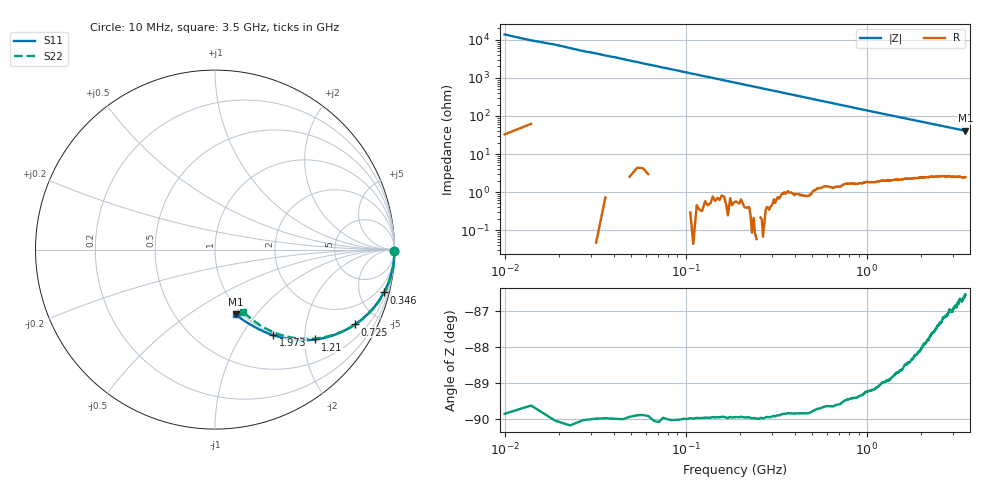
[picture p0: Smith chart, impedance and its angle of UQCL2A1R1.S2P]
! AVX Corporation
! Date:  10/27/06
! Part No:  UQCL2A1R1
! Description:  Ultra Low ESR Microwave capacitors
! Mounting Orientation:  Horizontal
# GHZ S DB R 50
! Freq  |S11|  S11 Ph  |S21|  S21 Ph  |S12|  S12 Ph  |S22|  S22 Ph
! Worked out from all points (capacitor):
!   801 points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, 10 MHz to 3.5 GHz, reference 50 ohm
!   read as one part in series: C = 1.13 pF near 27 MHz
!   lowest |Z| = 40.9 ohm at 3.5 GHz (marker M1)
!   S11 on the Smith chart (normalised r, x): 10 MHz: open; 346 MHz: 0.96, -7.89; 725 MHz: 0.98, -3.76; 1.21 GHz: 0.98, -2.25; 1.973 GHz: 0.98, -1.39; 3.5 GHz: 0.94, -0.79
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0.01  -0.01 -0.3  -42.87 89.5  -42.77 89.8  -0.01 -0.5
0.019  -0.01 -0.8  -37.53 89.3  -37.50 89.0  -0.01 -0.8
0.036  -0.01 -1.6  -31.81 88.4  -31.79 88.5  -0.01 -1.5
0.049  -0.01 -2.1  -29.15 87.9  -29.10 88.0  -0.01 -2.0
0.062  -0.01 -2.6  -27.09 87.3  -27.06 87.4  -0.01 -2.6
0.075  -0.01 -3.2  -25.44 86.8  -25.40 86.9  -0.01 -3.1
0.11  -0.02 -4.6  -22.13 85.4  -22.11 85.4  -0.01 -4.5
0.158  -0.05 -6.6  -19.03 83.4  -19.00 83.4  -0.02 -6.5
0.206  -0.10 -8.6  -16.77 81.4  -16.74 81.4  -0.06 -8.5
0.267  -0.15 -11.1  -14.57 79.0  -14.55 78.9  -0.12 -10.9
0.346  -0.26 -14.2  -12.43 75.7  -12.41 75.7  -0.22 -14.0
0.459  -0.45 -18.7  -10.16 71.3  -10.13 71.3  -0.41 -18.4
0.595  -0.74 -23.6  -8.20 66.2  -8.17 66.1  -0.70 -23.3
0.725  -1.06 -28.1  -6.79 61.6  -6.77 61.6  -1.03 -27.7
0.93  -1.64 -34.5  -5.22 55.1  -5.20 55.1  -1.61 -34.0
1.175  -2.38 -41.0  -3.97 48.5  -3.95 48.5  -2.36 -40.3
1.21  -2.49 -41.8  -3.83 47.6  -3.81 47.6  -2.47 -41.0
1.755  -4.16 -52.6  -2.38 36.9  -2.36 36.8  -4.16 -51.1
1.973  -4.80 -55.9  -2.06 33.6  -2.04 33.6  -4.80 -54.0
2.34  -5.78 -60.6  -1.68 29.2  -1.66 29.2  -5.79 -57.8
2.92  -7.16 -66.8  -1.33 24.2  -1.31 24.2  -7.18 -62.3
3.5  -8.44 -72.4  -1.14 20.6  -1.11 20.5  -8.38 -65.4
